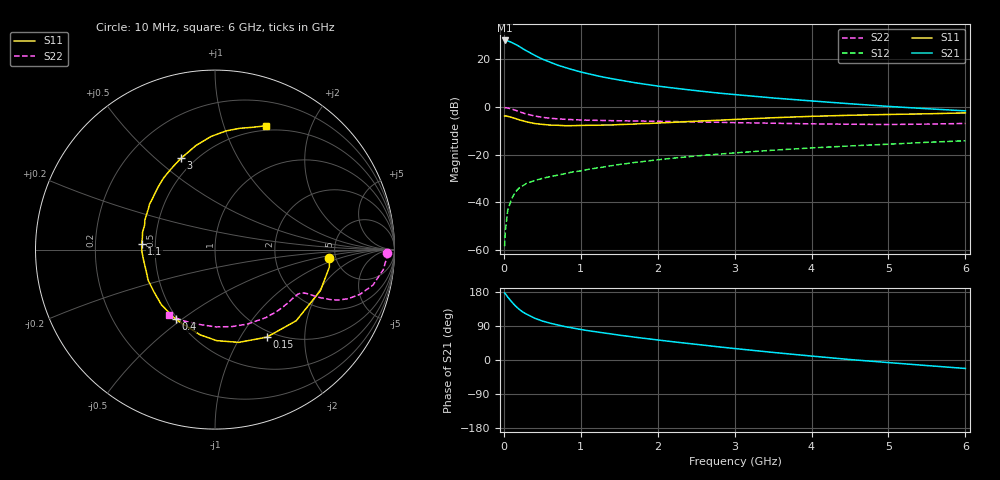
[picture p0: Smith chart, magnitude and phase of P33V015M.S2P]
! SIEMENS Small Signal Semiconductors
! BFP181
! Si NPN RF Bipolar Junction Transistor in SOT143
! VCE = 3 V  IC = 15 mA
! Common Emitter S-Parameters:  March  1996
# GHz  S  MA  R  50
!  f  S11  S21  S12  S22
! GHz  MAG  ANG  MAG  ANG  MAG  ANG  MAG  ANG
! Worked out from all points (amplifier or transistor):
!   36 points, 10 MHz to 6 GHz, reference 50 ohm
!   highest |S21| = 27.8 dB at 10 MHz (marker M1)
!   |S21| within 3 dB of that: start of sweep to 224.4 MHz
!   unconditionally stable (mu >= 1): 716.6 MHz to end of sweep
!   at 250 MHz: K = 0.49, MSG = 28.7 dB, |S12| = -33.0 dB
!   at 1.4 GHz: K = 1.25, MAG = 15.3 dB, |S12| = -24.7 dB
!   at 6 GHz: K = 1.02, MAG = 5.5 dB, |S12| = -14.2 dB
!   S11 on the Smith chart (normalised r, x): 10 MHz: 4.42, -0.72; 150 MHz: 0.91, -1.31; 400 MHz: 0.49, -0.47; 1.1 GHz: 0.42, +0.03; 3 GHz: 0.42, +0.61; 6 GHz: 0.45, +1.39
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0.01  0.639 -4.3  24.55 177.1  0.0012 94.4  0.9583 -1.1
0.02  0.6446 -8.7  24.49 174.7  0.0025 90.7  0.9584 -2.6
0.05  0.6303 -21.2  24.05 166.3  0.0067 83.5  0.9443 -6.8
0.1  0.6016 -41.2  22.35 153.9  0.0117 70.8  0.9017 -12.7
0.15  0.5668 -59.4  20.4 142.8  0.0164 64.8  0.8459 -17.1
0.2  0.5336 -75.6  18.41 133.7  0.02 60.1  0.79 -20.3
0.25  0.5074 -88.9  16.36 126.2  0.0223 57.1  0.741 -22.3
0.3  0.4821 -99.9  14.73 120.5  0.0252 54.9  0.7018 -23.4
0.4  0.4462 -119.5  12.02 110.3  0.0284 52.0  0.6423 -24.6
0.5  0.4285 -134.2  9.997 102.9  0.0316 51.1  0.602 -25.1
0.6  0.4137 -145.4  8.626 97.3  0.0343 51.4  0.5758 -25.4
0.7  0.4099 -155.2  7.456 92.4  0.0369 51.8  0.5586 -25.8
0.9  0.4023 -171.5  5.943 84.3  0.0432 52.8  0.5372 -26.9
1.1  0.41 175.8  4.919 77.2  0.0489 53.5  0.5238 -28.4
1.3  0.415 166.5  4.165 71.4  0.0548 53.7  0.5161 -30.6
1.6  0.4289 152.7  3.417 63.0  0.0646 53.3  0.507 -34.1
2.2  0.4725 131.8  2.478 48.1  0.0838 50.9  0.4903 -43.0
3  0.5428 110.4  1.806 30.3  0.1081 46.0  0.465 -56.8
3.5  0.5895 100.4  1.53 20.0  0.1231 42.4  0.4521 -66.7
4.5  0.6645 84.6  1.157 1.2  0.1512 34.5  0.4308 -89.4
5.5  0.7125 73.0  0.911 -14.7  0.1801 26.9  0.4334 -113.2
6  0.7449 67.8  0.822 -22.3  0.1941 22.6  0.4476 -125.2
